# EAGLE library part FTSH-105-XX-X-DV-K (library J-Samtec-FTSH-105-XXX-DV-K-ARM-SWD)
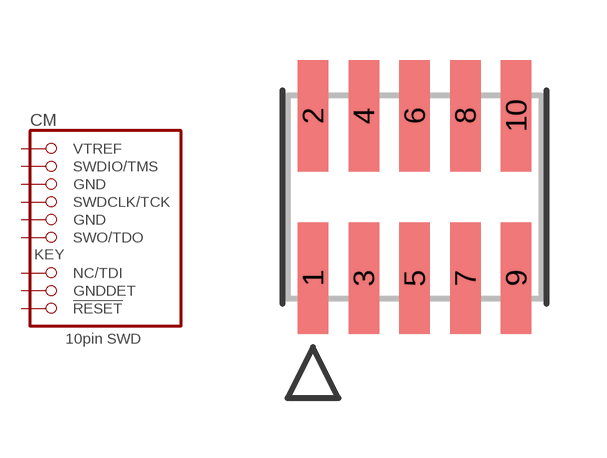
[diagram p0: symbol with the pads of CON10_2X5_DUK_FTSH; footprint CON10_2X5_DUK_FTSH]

Designator prefix CM

## FTSH-105-XX-X-DV-K  [CON10_2X5_DUK_FTSH]
1  VTREF  pas
2  SWDIO/TMS  pas
3  GND  pas
4  SWDCLK/TCK  pas
5  GND  pas
6  SWO/TDO  pas
8  NC/TDI  pas
9  GNDDET  pas
10  !RESET  pas

## Footprint CON10_2X5_DUK_FTSH (pad centres in mm)
smd 0.762 x 2.794: 1 -2.54,-2.032; 2 -2.54,2.032; 3 -1.27,-2.032; 4 -1.27,2.032; 5 0,-2.032; 6 0,2.032; 7 1.27,-2.032; 8 1.27,2.032; 9 2.54,-2.032; 10 2.54,2.032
